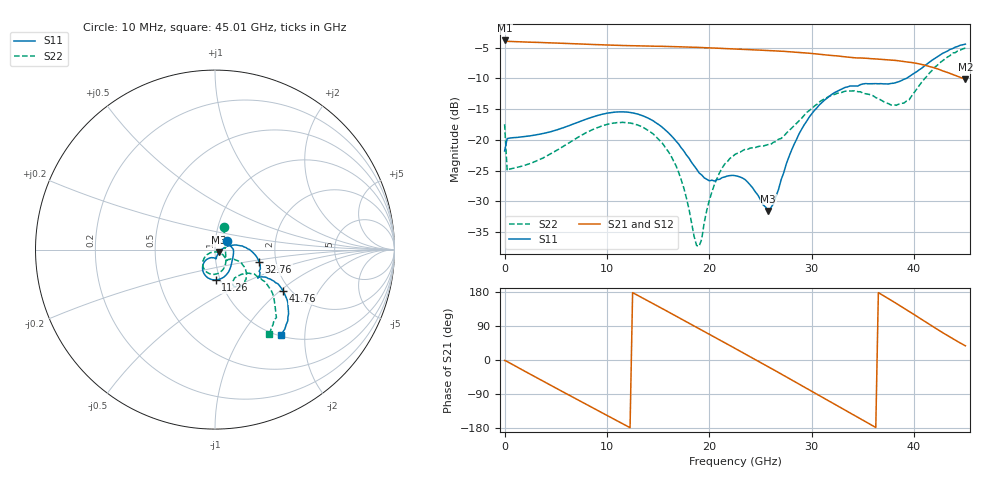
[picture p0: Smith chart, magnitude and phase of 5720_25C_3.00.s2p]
! Device:  ADRF5720
! Description: 0.5dB LSB GaAs MMIC 6-bit Digital Attenuator
! Frequency:  0.000009 -  40 GHz
! Ports:
!	RF1	= Port 1
!	RF2	= Port 2
! Vdd:  3.3 Volt
! Vss:  -3.3 Volt
! Control:  0/3.3 Volt
! State:  3.00 dB attenuation
! Data:  The device was measured using G-S-G Probes on a matrix board.
!  Data was collected using an calibrated 4 port network analyzer.
!  The reference plane for this measurement is at the launchers.
! Note:  Analog Devices supplies this data as a sample of measured data
!  for this product.  Your particular data for this product may vary.
!  Data was taken at 25 degrees C.
!  Analog Devices reserves the right to change this data at anytime.
# GHZ S DB R 45.0
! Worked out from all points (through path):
!   181 points, 10 MHz to 45.01 GHz, reference 45 ohm
!   highest |S21| = -3.82 dB at 10 MHz (marker M1); lowest = -10.1 dB at 45.01 GHz (marker M2)
!   group delay of S21, straight-line fit = 41.8 ps
!   lowest |S11| = -31.6 dB at 25.76 GHz (marker M3), VSWR 1.05, Z = 46.9 - j1.48 ohm
!   |S11| at or under -10 dB: start of sweep to 39.24 GHz
!   |S22| runs from -37.3 to -5.1 dB; largest |S21 - S12| = 0.00075
!   S11 on the Smith chart (normalised r, x): 10 MHz: 1.14, +0.11; 11.26 GHz: 0.95, -0.33; 32.76 GHz: 1.63, -0.24; 41.76 GHz: 1.83, -1.06; 45.01 GHz: 1.03, -1.52
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0.01  -21.81 35.3  -3.82 -1.2  -3.82 -1.2  -17.46 68.0
0.26  -19.80 0.5  -3.96 -4.1  -3.96 -4.1  -25.00 2.6
2.01  -19.46 -16.8  -4.07 -30.1  -4.07 -30.1  -24.12 -18.0
4.26  -18.78 -34.3  -4.20 -63.0  -4.20 -63.0  -22.51 -36.5
7.76  -16.76 -58.6  -4.42 -113.8  -4.41 -113.8  -19.02 -62.3
11.26  -15.45 -88.5  -4.63 -164.2  -4.62 -164.2  -17.19 -94.5
13.26  -15.95 -106.7  -4.71 166.9  -4.71 166.9  -17.76 -115.0
15.26  -17.76 -122.2  -4.77 137.8  -4.77 137.8  -20.27 -134.5
17.01  -20.69 -130.7  -4.85 112.1  -4.85 112.2  -25.32 -147.3
18.76  -24.77 -124.0  -4.94 86.3  -4.94 86.3  -37.21 -102.0
19.01  -25.40 -121.3  -4.96 82.6  -4.96 82.6  -37.31 -73.3
20.51  -26.71 -97.9  -5.06 60.4  -5.06 60.4  -27.22 -31.3
22.76  -25.92 -83.0  -5.23 27.0  -5.23 27.0  -22.18 -40.3
25.76  -31.60 -36.9  -5.46 -17.8  -5.46 -17.8  -20.76 -39.1
28.26  -20.81 14.8  -5.70 -55.9  -5.70 -55.9  -17.74 -26.5
30.26  -15.23 3.7  -5.98 -86.5  -5.98 -86.5  -14.51 -30.4
32.76  -11.87 -15.4  -6.39 -124.5  -6.39 -124.5  -12.38 -46.0
35.51  -10.87 -31.1  -6.74 -166.4  -6.74 -166.4  -12.56 -61.2
37.76  -10.81 -32.6  -7.01 157.6  -7.01 157.7  -14.34 -55.5
39.51  -9.71 -28.4  -7.37 128.3  -7.37 128.4  -13.49 -38.5
41.76  -7.03 -31.4  -8.17 89.6  -8.17 89.7  -8.69 -35.0
45.01  -4.42 -52.0  -10.14 37.4  -10.14 37.4  -5.06 -57.2
